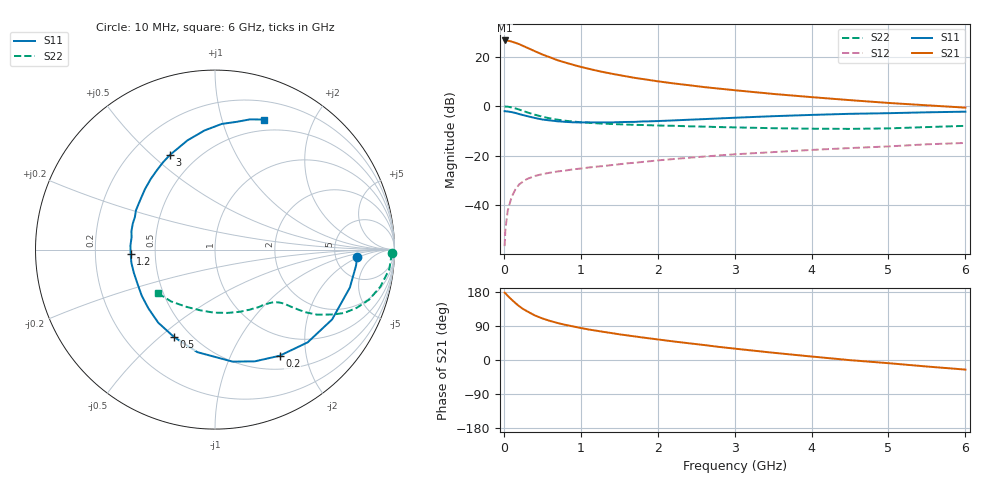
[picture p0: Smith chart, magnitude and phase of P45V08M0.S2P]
! SIEMENS Small Signal Semiconductors
! BFP182
! Si NPN RF Bipolar Junction Transistor in SOT143
! VCE = 5 V  IC = 8 mA
! Common Emitter S-Parameters:  March  1996
# GHz  S  MA  R  50
!  f  S11  S21  S12  S22
! GHz  MAG  ANG  MAG  ANG  MAG  ANG  MAG  ANG
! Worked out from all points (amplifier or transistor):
!   36 points, 10 MHz to 6 GHz, reference 50 ohm
!   highest |S21| = 26.5 dB at 10 MHz (marker M1)
!   |S21| within 3 dB of that: start of sweep to 307.9 MHz
!   unconditionally stable (mu >= 1): 1.325 GHz to 5.447 GHz
!   at 250 MHz: K = 0.27, MSG = 27.4 dB, |S12| = -30.4 dB
!   at 1.4 GHz: K = 1.03, MAG = 17.5 dB, |S12| = -23.8 dB
!   at 6 GHz: K = 0.94, MSG = 7.1 dB, |S12| = -14.8 dB
!   lowest NFmin = 1.40 dB at 450 MHz
!   S11 on the Smith chart (normalised r, x): 10 MHz: 8.17, -1.88; 200 MHz: 0.68, -1.56; 500 MHz: 0.41, -0.56; 1.2 GHz: 0.36, -0.02; 3 GHz: 0.36, +0.57; 6 GHz: 0.38, +1.38
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0.01  0.7919 -3.1  21.16 177.8  0.0015 83.2  0.9856 -1.2
0.02  0.791 -6.4  21.06 176.1  0.0032 90.0  0.9825 -2.6
0.05  0.7807 -15.7  20.95 169.5  0.0077 85.5  0.9769 -6.5
0.1  0.7597 -30.8  20.12 159.6  0.0146 74.4  0.9445 -12.6
0.15  0.7306 -45.0  18.97 150.3  0.0209 67.9  0.9025 -18.0
0.2  0.6924 -58.7  17.84 141.9  0.0265 63.1  0.8531 -22.4
0.25  0.6609 -70.4  16.42 134.7  0.0302 58.5  0.802 -26.1
0.3  0.6318 -81.1  15.17 128.9  0.0339 54.7  0.7526 -28.7
0.4  0.5798 -99.7  12.92 117.9  0.039 48.7  0.6748 -32.5
0.5  0.5385 -114.9  11.04 109.7  0.0426 45.2  0.6133 -34.7
0.6  0.5156 -127.8  9.672 103.1  0.0455 43.6  0.5667 -35.9
0.7  0.495 -138.5  8.438 97.6  0.0483 42.5  0.5333 -36.8
0.9  0.4723 -155.7  6.839 88.6  0.0533 41.3  0.4894 -38.0
1.1  0.4717 -171.1  5.701 80.6  0.0578 41.0  0.4621 -39.6
1.2  0.4706 -177.2  5.236 77.4  0.0602 40.8  0.4516 -40.5
1.7  0.4819 157.8  3.729 62.3  0.0722 41.2  0.4206 -45.7
2.2  0.5156 139.1  2.888 49.1  0.0856 39.9  0.4022 -53.0
3  0.5843 115.4  2.099 30.0  0.1068 36.0  0.3738 -67.9
3.5  0.6278 104.1  1.767 19.2  0.1184 32.8  0.3594 -78.9
4.5  0.7013 86.9  1.323 -0.4  0.1429 26.3  0.3482 -104.2
5.5  0.7516 74.9  1.041 -17.2  0.1702 19.6  0.3785 -130.2
6  0.7748 69.2  0.934 -25.3  0.1813 15.0  0.4007 -142.8
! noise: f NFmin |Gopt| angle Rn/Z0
0.45  1.4  0.26  41  0.29
0.9  1.5  0.25  83  0.23
1.8  2  0.21  162  0.2
